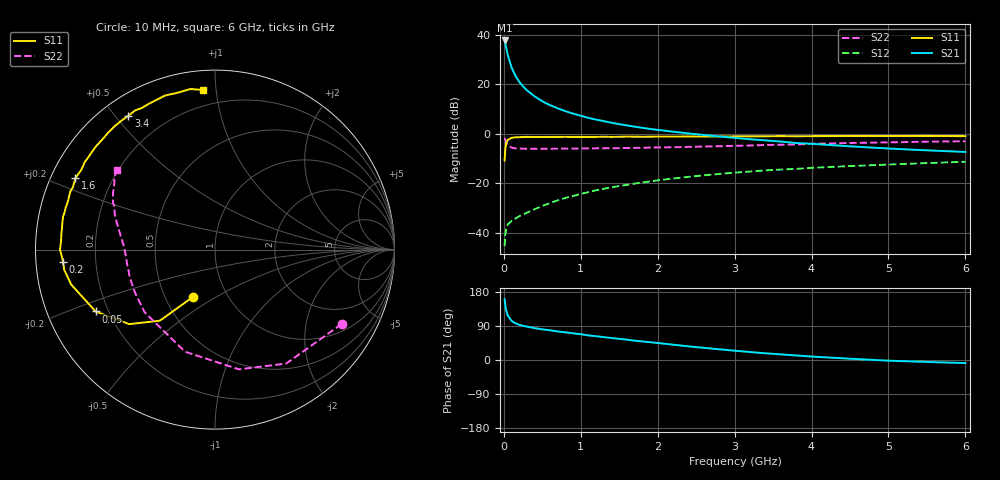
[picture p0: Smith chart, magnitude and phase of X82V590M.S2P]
! SIEMENS Small Signal Semiconductors
! BFP136W
! Si NPN RF Bipolar Junction Transistor in SOT343
! VCE = 2.5 V  IC = 90 mA
! Common Emitter S-Parameters:  September  1994
# GHz  S  MA  R  50
!  f  S11  S21  S12  S22
! GHz  MAG  ANG  MAG  ANG  MAG  ANG  MAG  ANG
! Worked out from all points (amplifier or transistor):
!   40 points, 10 MHz to 6 GHz, reference 50 ohm
!   highest |S21| = 37.8 dB at 10 MHz (marker M1)
!   |S21| within 3 dB of that: start of sweep to 31.28 MHz
!   unconditionally stable (mu >= 1): 494.1 MHz to 2.888 GHz
!   at 200 MHz: K = 0.69, MSG = 27.2 dB, |S12| = -33.4 dB
!   at 1.5 GHz: K = 1.10, MAG = 10.6 dB, |S12| = -21.2 dB
!   at 6 GHz: K = 0.97, MSG = 2.0 dB, |S12| = -11.3 dB
!   S11 on the Smith chart (normalised r, x): 10 MHz: 0.69, -0.40; 50 MHz: 0.15, -0.24; 200 MHz: 0.08, -0.04; 1.6 GHz: 0.07, +0.24; 3.4 GHz: 0.08, +0.54; 6 GHz: 0.11, +0.92
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0.01  0.2882 -114.7  77.22 160.2  0.0053 67.6  0.8186 -30.4
0.02  0.5013 -127.8  66.49 143.7  0.0095 58.6  0.7487 -58.0
0.03  0.633 -139.0  55.86 132.0  0.0118 48.0  0.6804 -78.7
0.05  0.749 -152.6  39.82 117.9  0.0145 38.5  0.5928 -106.4
0.1  0.8242 -166.3  22 103.3  0.0172 34.8  0.5252 -138.3
0.15  0.8476 -172.3  14.96 96.9  0.0192 39.0  0.5062 -151.5
0.2  0.85 -175.5  11.22 93.0  0.0214 41.0  0.5001 -158.6
0.25  0.8567 -178.2  9.052 90.1  0.0232 45.2  0.4983 -163.1
0.3  0.8637 180.0  7.569 88.0  0.0252 48.4  0.4959 -166.2
0.4  0.8587 176.7  5.698 84.1  0.0297 52.8  0.4965 -170.2
0.5  0.8608 174.0  4.543 80.9  0.0346 55.5  0.4962 -172.9
0.6  0.861 172.0  3.789 78.4  0.0395 58.0  0.4974 -174.7
0.7  0.8641 169.5  3.268 75.3  0.0448 60.1  0.4985 -176.0
0.9  0.8632 166.1  2.555 70.4  0.055 61.3  0.5008 -178.6
1.1  0.8622 161.7  2.091 64.9  0.0659 61.7  0.5046 179.8
1.6  0.8732 152.9  1.47 53.8  0.0922 60.2  0.5152 175.9
2.2  0.874 142.9  1.098 40.4  0.1239 55.7  0.5324 171.3
3.2  0.8875 125.9  0.773 21.1  0.1717 46.2  0.5782 162.5
3.4  0.8884 122.9  0.734 17.7  0.1812 44.1  0.5915 160.7
4.5  0.9023 108.0  0.556 3.4  0.2217 33.7  0.6501 150.9
5.5  0.9053 98.7  0.461 -5.1  0.2547 25.7  0.6901 144.1
6  0.8919 94.4  0.428 -8.1  0.2708 21.3  0.7051 141.1
